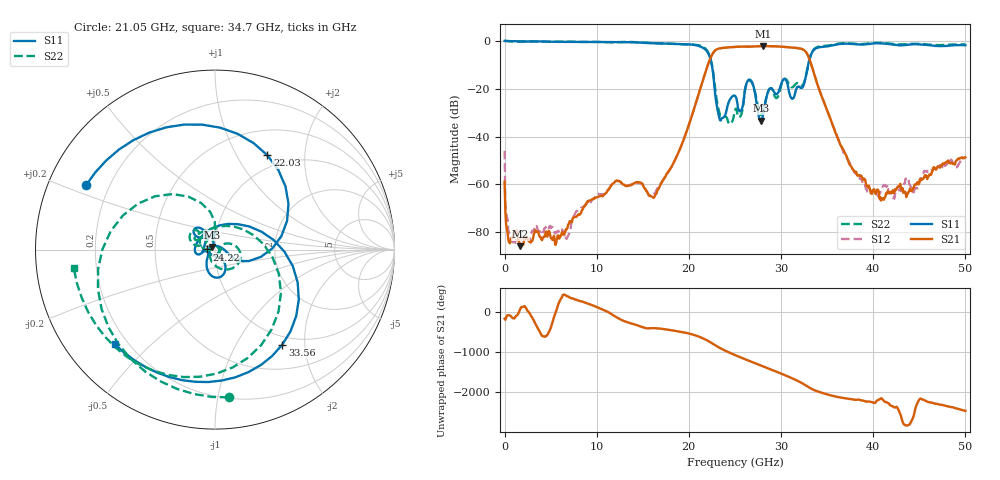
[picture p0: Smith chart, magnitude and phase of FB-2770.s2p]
! MARKI MICROWAVE INC.
! Email:  info@markimicrowave.com  Phone:  408-778-4200
! Model Number:  FB-2770  Date:  03/12
! Filename:		FB-2770.S2P  Version: 1.0
! Description:  2-port S-parameter data for Band Pass Filter FB-2770
! Frequency Measured: 	10 MHz to 50 GHz
! Measurements:		S11, S21, S12, S22
# Hz S  dB  R 50
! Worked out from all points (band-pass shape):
!   617 points, 10 MHz to 50.05 GHz, reference 50 ohm
!   highest |S21| = -2.01 dB at 28.12 GHz (marker M1); lowest = -86.0 dB at 1.716 GHz (marker M2)
!   |S21| within 3 dB of the highest: 22.63 GHz to 32.82 GHz (10.19 GHz wide, 36.8 % of centre)
!   lowest |S11| = -33.4 dB at 27.87 GHz (marker M3), VSWR 1.04, Z = 48.5 + j1.44 ohm
!   |S11| at or under -10 dB: 22.52 GHz to 32.97 GHz (10.45 GHz wide, 37.7 % of centre)
!   |S22| runs from -34.7 to 0.3 dB; largest |S21 - S12| = 0.0056
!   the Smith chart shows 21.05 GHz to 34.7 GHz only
!   S11 on the Smith chart (normalised r, x): 21.05 GHz: 0.12, +0.23; 22.03 GHz: 0.82, +1.35; 24.22 GHz: 0.92, +0.00; 33.56 GHz: 0.86, -1.58; 34.7 GHz: 0.15, -0.39
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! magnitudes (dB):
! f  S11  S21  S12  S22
! 10 MHz  0.2  -59.0  -45.9  0.3
! 497.4 MHz  0.1  -84.3  -81.5  0.0
! 1.716 GHz  0.0  -86.0  -82.6  -0.1
! 8.377 GHz  -0.2  -71.1  -69.8  -0.3
! 12.2 GHz  -0.4  -58.5  -58.5  -0.4
! 16.74 GHz  -0.9  -61.8  -61.0  -0.9
! 21.05 GHz  -1.9  -22.5  -22.5  -1.7
! 22.03 GHz  -4.4  -10.6  -10.6  -4.0
! 23.33 GHz  -32.1  -3.0  -3.0  -29.9
! 24.22 GHz  -27.1  -2.6  -2.6  -32.9
! 25.03 GHz  -22.9  -2.4  -2.4  -28.9
! 25.68 GHz  -29.1  -2.2  -2.2  -31.0
! 26.57 GHz  -16.1  -2.3  -2.3  -16.4
! 27.87 GHz  -33.4  -2.0  -2.0  -31.0
! 28.12 GHz  -30.1  -2.0  -2.0  -29.1
! 32.34 GHz  -19.4  -3.3  -3.3  -18.5
! 33.4 GHz  -4.7  -10.8  -10.8  -4.6
! 33.56 GHz  -3.8  -12.9  -12.9  -3.6
! 34.7 GHz  -2.3  -25.6  -25.6  -2.0
! 39.49 GHz  -1.2  -61.4  -63.4  -0.9
! 41.77 GHz  -1.2  -63.8  -63.4  -0.9
! 50.05 GHz  -1.6  -48.7  -49.1  -1.3
